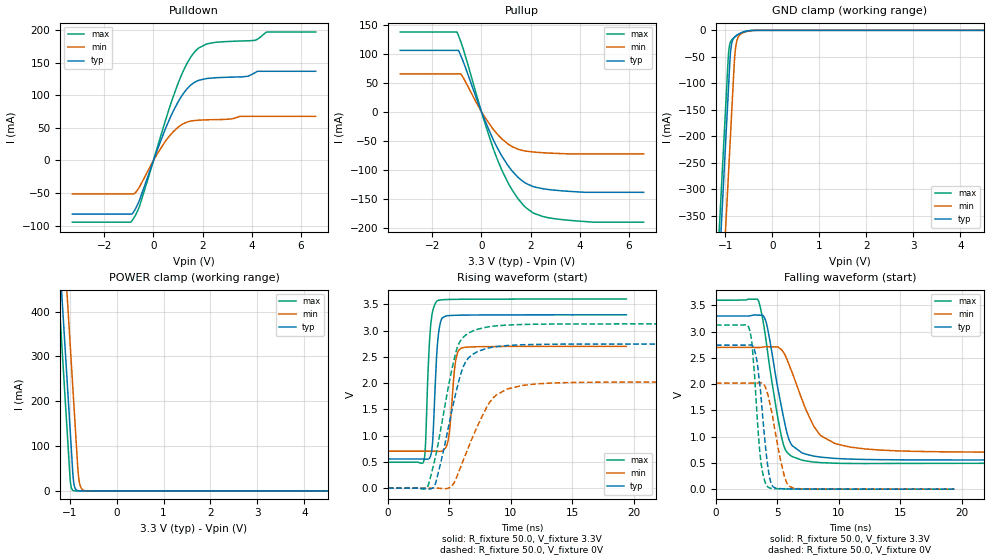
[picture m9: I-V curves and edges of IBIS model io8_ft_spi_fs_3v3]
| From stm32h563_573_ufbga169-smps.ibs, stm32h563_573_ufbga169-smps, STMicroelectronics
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[Model]   io8_ft_spi_fs_3v3
Model_type I/O
Polarity   Non-Inverting
Enable   Active-Low
| CAP_THRESHOLD on pad IOFT is "UDTCAPC" :
| Rising=20.0% of vddiom   Falling=80.0% of vddiom
| C_comp min and max val. don't necessarily correlate with the min and max pvt
| but are the smallest and greatest pad capacitance found.
| var   typ   min   max
C_comp   5.03687pF  4.97386pF  5.04450pF
|C_comp_pullup   3.26850pF  3.10785pF  3.04350pF
|C_comp_pulldown   1.76837pF  1.86601pF  2.00100pF
Vinl = 810.0mV
Vinh = 2.52V
Vmeas = 1.65V   | Reference voltage for timing measurements
Cref  = 50.0pF   | Timing specification test load capacitance value
Rref  = 100.0MOhm   | Timing specification test load resistance value
Vref  = 1.65V   | Timing specification test load voltage
[Model Spec]
| TIME_THRESHOLD on pin ZIV11 is "CMOS" :
| Rising=40.0% of vdd   Falling=60.0% of vdd
Vinl 1.29880V 1.07480V 1.40680V
Vinh 1.77520V 1.49320V 1.89720V
| variable   typ   min   max
[Temperature Range] 25.0 125.0 -40.0
| variable   typ   min   max
[Voltage Range] 3.3V 2.7V 3.6V
| variable   typ   min   max
[POWER Clamp Reference] 3.3V 2.7V 3.6V
| variable   typ   min   max
[GND Clamp Reference] 0V 0V 0V
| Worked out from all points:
|   slope of the pulldown table from 0 to 0.495 V, typ, clamps not added: 10 ohm
|   slope of the pullup table from 0 to 0.495 V, typ, clamps not added: 10 ohm
|   GND clamp passes 1 mA (typ) near -0.52 V on its own axis
|   POWER clamp passes 1 mA (typ) near -0.84 V on its own axis
|   rising waveform, R_fixture 50.0, V_fixture 3.3V: 20-80 % time 343ps typ, 423ps min, 333ps max; typ from 0.556 V to 3.3 V
|   falling waveform, R_fixture 50.0, V_fixture 3.3V: 20-80 % time 1.3ns typ, 2.19ns min, 1.25ns max; typ from 3.3 V to 0.556 V
|   rising waveform, R_fixture 50.0, V_fixture 0V: 20-80 % time 1.6ns typ, 2.31ns min, 1.55ns max; typ from 0 V to 2.74 V
|   falling waveform, R_fixture 50.0, V_fixture 0V: 20-80 % time 689ps typ, 1.01ns min, 581ps max; typ from 2.74 V to 0 V
[POWER Clamp]
-3.3V     4.068A     4.259A     3.957A
-1.25V    582.8mA    774.2mA    471.5mA
-1.13V    378.8mA    570.2mA    267.5mA
-1.09V    310.8mA    502.2mA    199.5mA
-1.02V    191.8mA    383.2mA    80.53mA
-990mV    140.8mA    332.2mA    29.53mA
-920mV    26.3mA     213.2mA    906uA
-880mV    5.543mA    145.2mA    123.7uA
-810mV    363.5uA    33.6mA     3.798uA
-770mV    76.62uA    10.47mA    519.4nA
-690mV    3.409uA    1.017mA    10.48nA
6.6V      0A         0A         0A
[GND Clamp]
-3.3V     -4.131A    -4.293A    -4.064A
-1.25V    -646.2mA   -808mA     -579.5mA
-940mV    -119.2mA   -281mA     -52.48mA
-920mV    -85.23mA   -247mA     -32.7mA
-900mV    -51.91mA   -213mA     -24.27mA
-870mV    -26.87mA   -162mA     -18.7mA
-810mV    -13.22mA   -60.41mA   -13.31mA
-790mV    -11.41mA   -38.37mA   -11.93mA
-740mV    -8.18mA    -15.37mA   -8.882mA
-660mV    -4.605mA   -6.274mA   -4.919mA
-320mV    -10.56uA   -77.76uA   -2.038uA
6.6V      9.514nA    1.879uA    704.5pA
| variable   typ   min   max
[Pullup Reference] 3.3V 2.7V 3.6V
| variable   typ   min   max
[Pulldown Reference] 0V 0V 0V
[Pullup]
-3.3V     105.6mA    65.02mA    137.2mA
-990mV    105.6mA    65.02mA    137.2mA
-930mV    105.6mA    65.02mA    130.9mA
-830mV    95.8mA     65.02mA    119.6mA
120mV     -12.96mA   -8.365mA   -16.99mA
680mV     -65.11mA   -40.43mA   -85.66mA
1.26V     -102.9mA   -60.65mA   -135.8mA
1.83V     -124.2mA   -68.3mA    -166.4mA
2.51V     -133.2mA   -71mA      -181.1mA
3.19V     -136.4mA   -72.38mA   -186mA
4.54V     -139.3mA   -72.9mA    -190.8mA
6.6V      -139.3mA   -72.9mA    -190.8mA
[Pulldown]
-3.3V     -82.43mA   -51.49mA   -94.82mA
-860mV    -81.66mA   -51.49mA   -91.78mA
-560mV    -60.16mA   -40.13mA   -69.41mA
120mV     12.61mA    7.999mA    15.37mA
800mV     75.3mA     43.94mA    97.52mA
1.33V     108.3mA    58.37mA    146.5mA
1.84V     123.1mA    61.83mA    172.7mA
2.51V     126.9mA    62.7mA     181.3mA
3.84V     129.3mA    67.77mA    183.7mA
4.13V     134.7mA    67.77mA    184.6mA
4.59V     136.9mA    67.77mA    197.1mA
6.6V      136.9mA    67.77mA    197.1mA
[Ramp]
dV/dt_r 1.64629V/1.59508ns 1.21235V/2.31384ns 1.87635V/1.54426ns
dV/dt_f 1.64666V/1.30073ns 1.19801V/2.15021ns 1.86387V/1.24494ns
R_load = 50.0
| Removed startup time: 0s 0s 0s  .
| Removed end time: 19.4ns.
[Rising Waveform]
R_fixture   = 50.0
V_fixture   = 3.3V
V_fixture_min = 2.7V
V_fixture_max = 3.6V
0s        555.6mV    703.3mV    493.6mV
2.9ns     555.4mV    703.3mV    509.4mV
3.05ns    552.2mV    703.3mV    832.4mV
3.35ns    565.6mV    703.3mV    2.694V
3.6ns     798.9mV    703.3mV    3.333V
4ns       2.685V     701.6mV    3.565V
4.85ns    3.283V     869.3mV    3.592V
5.5ns     3.291V     2.417V     3.595V
5.95ns    3.294V     2.667V     3.596V
19.4ns    3.3V       2.7V       3.6V
| Removed startup time: 0s 0s 0s  .
| Removed end time: 59.4ns.
[Falling Waveform]
R_fixture   = 50.0
V_fixture   = 3.3V
V_fixture_min = 2.7V
V_fixture_max = 3.6V
0s        3.3V       2.7V       3.6V
3.45ns    3.316V     2.699V     3.594V
4.1ns     3.168V     2.714V     2.793V
4.9ns     2.1V       2.71V      1.54V
5.45ns    1.427V     2.623V     886.3mV
6.05ns    888.4mV    2.313V     644.7mV
7ns       692mV      1.71V      552.7mV
8.5ns     611.1mV    1.024V     506.2mV
12.2ns    565.7mV    764.9mV    488.6mV
59.4ns    555.6mV    703.3mV    493.6mV
| Removed startup time: 0s 0s 0s  .
| Removed end time: 59.4ns.
[Rising Waveform]
R_fixture   = 50.0
V_fixture   = 0V
V_fixture_min = 0V
V_fixture_max = 0V
0s        103.7nV    446.5nV    93.92nV
3.1ns     -5mV       -521.2nV   -7.245mV
3.7ns     17.23mV    239.2uV    439.1mV
5ns       1.259V     11.46mV    2.036V
5.7ns     1.985V     279.5mV    2.719V
6.5ns     2.464V     751.5mV    2.943V
8ns       2.659V     1.53V      3.065V
9.7ns     2.716V     1.887V     3.105V
13.4ns    2.741V     2.003V     3.124V
59.4ns    2.744V     2.021V     3.127V
| Removed startup time: 0s 0s 0s  .
| Removed end time: 19.4ns.
[Falling Waveform]
R_fixture   = 50.0
V_fixture   = 0V
V_fixture_min = 0V
V_fixture_max = 0V
0s        2.744V     2.021V     3.127V
2.7ns     2.746V     2.021V     3.059V
2.95ns    2.74V      2.021V     2.723V
3.2ns     2.596V     2.021V     1.955V
3.65ns    1.811V     2.028V     536.6mV
4.25ns    383.9mV    1.774V     37.7mV
4.65ns    47.79mV    1.328V     11.77mV
5.3ns     9.759mV    505mV      5.559mV
5.95ns    5.618mV    56.39mV    3.433mV
19.4ns    37.38uV    108.8uV    44.76uV
